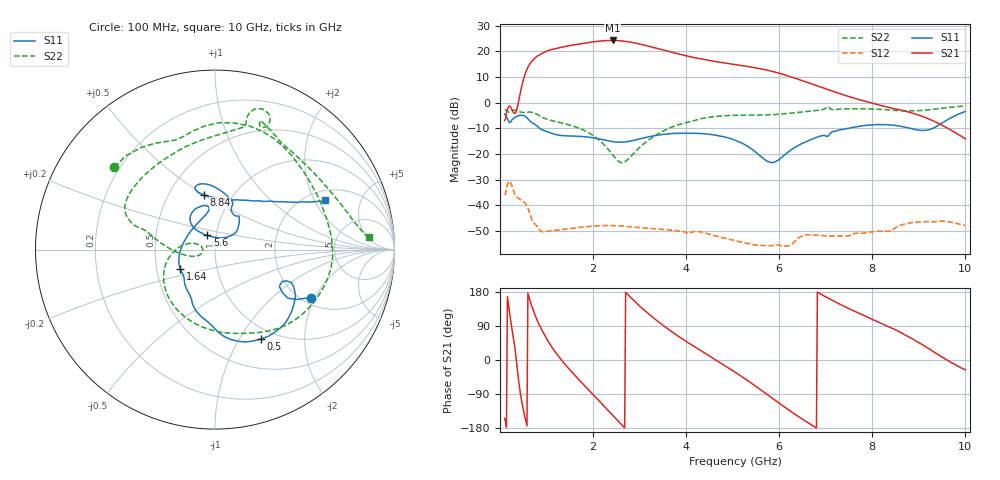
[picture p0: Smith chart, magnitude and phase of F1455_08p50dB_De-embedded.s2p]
! Integrated Device Technology
! Corporate Headquarters
! 6024 Silver Creek Valley Road
! San Jose, CA 95138  USA
! Phone:  1-408-284-8200
! Toll Free:  1-800-223-1366
! Webpage:  http://www.idt.com/
! Timing and RF Division
! 515 Groton Road, Suite 102
! Westford, MA 01886-6024
! Device:  F1455
! Description: 6-bit 0.5 dB Transmit Variable Gain Amplifier
! Frequency:  1400.0 -  2300.00 MHz
! Package:  6x6 mm Thin QFN Plastic Package: 28 pin
! State:  17
! Atten State:  8.5 dB
! Voltage:  +5.00 Volts
! Current:  217.679 mA
! Data:  The device was measured on a the F1455 evaluation board which has
!  individual transmission lines to the RF pins.  Data was collected
!  using a calibrated network analyzer.  The evaluation board was
!  de-embedded using a TRL calibration technique.
!  The reference plane is the edge of the package pin.
!  Pin  1 = CSb
!  Pin  2 = DATA
!  Pin  3 = CLK
!  Pin  4 = RSET
!  Pin  5 = GND
!  Pin  6 = RFIN  = Port 1
!  Pin  7 = GND
!  Pin  8 = NC
!  Pin  9 = NC
!  Pin 10 = NC
!  Pin 11 = NC
!  Pin 12 = NC
!  Pin 13 = NC
!  Pin 14 = /STBY
!  Pin 15 = GND
!  Pin 16 = RFOUT  = Port 2
!  Pin 17 = GND
!  Pin 18 = NC
!  Pin 19 = NC
!  Pin 20 = NC
!  Pin 21 = GND
!  Pin 22 = NC
!  Pin 23 = GND
!  Pin 24 = NC
!  Pin 25 = NC
!  Pin 26 = NC
!  Pin 27 = GND
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# GHz S dB R 50
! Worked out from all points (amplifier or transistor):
!   496 points, 100 MHz to 10 GHz, reference 50 ohm
!   highest |S21| = 24.3 dB at 2.42 GHz (marker M1)
!   |S21| within 3 dB of that: 1.236 GHz to 3.355 GHz (2.118 GHz wide, 92.3 % of centre)
!   unconditionally stable (mu >= 1): start of sweep to end of sweep
!   at 1.74 GHz: K = 8.20, MAG = 23.7 dB, |S12| = -48.6 dB
!   at 5.06 GHz: K = 29.11, MAG = 16.7 dB, |S12| = -53.9 dB
!   at 10 GHz: K = 88.92, MAG = -5.6 dB, |S12| = -47.9 dB
!   S11 on the Smith chart (normalised r, x): 100 MHz: 2.22, -1.87; 500 MHz: 0.86, -1.24; 1.64 GHz: 0.66, -0.15; 5.6 GHz: 0.91, +0.15; 8.84 GHz: 0.74, +0.50; 10 GHz: 2.45, +2.44
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0.1  -4.44 -26.7  -6.94 -153.8  -36.10 44.2  -2.81 140.7
0.38  -5.21 -39.0  -1.32 -32.4  -37.16 -110.8  -3.26 56.3
0.5  -5.03 -62.7  8.77 -130.5  -38.62 -148.9  -3.80 28.3
0.68  -7.70 -94.4  16.03 143.5  -45.42 149.6  -3.76 -13.8
0.82  -9.52 -111.3  18.38 98.8  -48.86 132.1  -4.76 -46.5
0.96  -10.99 -121.3  19.80 65.7  -50.42 123.7  -6.14 -71.2
1.28  -12.76 -138.9  21.47 6.4  -49.67 86.8  -7.73 -114.0
1.64  -13.09 -151.1  22.73 -44.7  -48.87 54.6  -9.56 -149.2
1.76  -13.21 -155.6  23.09 -60.3  -48.56 45.5  -10.41 -159.2
2.1  -14.06 -173.0  23.96 -104.0  -48.09 22.4  -14.16 175.3
2.42  -15.19 159.6  24.29 -145.6  -47.97 2.2  -20.33 163.0
2.68  -15.33 132.0  23.98 -179.0  -48.25 -12.2  -23.09 -170.5
2.96  -14.35 109.5  23.08 147.2  -48.71 -25.6  -18.14 -162.3
3.4  -12.65 98.0  21.07 101.3  -49.34 -42.7  -12.17 179.3
3.74  -12.03 101.6  19.48 70.5  -49.93 -56.3  -9.23 168.9
4.1  -11.94 111.1  17.87 41.3  -50.66 -64.8  -7.37 164.0
5.06  -14.68 133.5  14.87 -32.7  -53.87 -102.9  -4.91 149.0
5.6  -20.91 118.1  13.23 -78.4  -55.77 -108.7  -4.85 127.6
6.7  -14.31 46.6  7.33 -171.9  -51.63 -140.5  -3.23 78.6
8.36  -8.66 106.7  -1.91 87.2  -50.17 164.9  -2.84 62.6
8.84  -10.13 101.7  -3.98 57.0  -46.86 148.4  -3.21 44.4
10  -3.45 24.0  -14.15 -26.0  -47.91 77.5  -1.29 4.7
